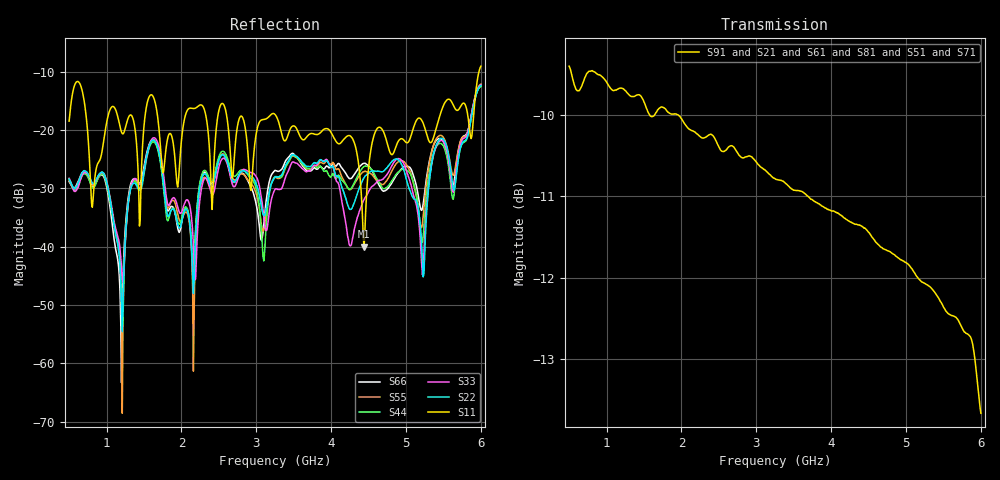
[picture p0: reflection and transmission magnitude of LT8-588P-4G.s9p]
! MTS Systemtechnik GmbH
! S-Parameters
! Model: LT8-588P-6G
! Rohde & Schwarz ZVB8 2Ports - Version 3.20 - 1145.1010k08 SN: 100119
! Converted & adapted with MATLAB
!		|  MTS  |
!		|  |--o OUT 8 (Port 9)
!		|  |--o OUT 7 (Port 8)
!		|  |--o OUT 6 (Port 7)
!		|  |--o OUT 5 (Port 6)
! C (Port 1) o--| LT8-588P-6G |
!		|  |--o OUT 4 (Port 5)
!		|  |--o OUT 3 (Port 4)
!		|  |--o OUT 2 (Port 3)
!		|  |--o OUT 1 (Port 2)
! S9P File: Measurements:
! <S11,S12,S13,S14,S15,S16,S17,S18,S19>,
! <S21,S22,S23,S24,S25,S26,S27,S28,S29>,
! <S31,S32,S33,S34,S35,S36,S37,S38,S39>,
! <S41,S42,S43,S44,S45,S46,S47,S48,S49>,
! <S51,S52,S53,S54,S55,S56,S57,S58,S59>,
! <S61,S62,S63,S64,S65,S66,S67,S68,S69>,
! <S71,S72,S73,S74,S75,S76,S77,S78,S79>,
! <S81,S82,S83,S84,S85,S86,S87,S88,S89>,
! <S91,S92,S93,S94,S95,S96,S97,S98,S99>:
# HZ  S  DB  R  50.00
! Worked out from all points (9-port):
!   551 points, 500 MHz to 6 GHz, reference 50 ohm
!   strongest paths, dB at 500 MHz, 1.87 GHz, 3.25 GHz, 4.63 GHz, 6 GHz:
!     S91: -9.4, -10.0, -10.8, -11.6, -13.7
!     S21: -9.4, -10.0, -10.8, -11.6, -13.8
!     S61: -9.4, -10.0, -10.8, -11.7, -13.7
!     S81: -9.4, -10.0, -10.8, -11.6, -13.8
!     S51: -9.4, -10.0, -10.8, -11.7, -13.8
!     S71: -9.4, -10.0, -10.8, -11.7, -13.7
!   lowest |S11| = -40.0 dB at 4.44 GHz (marker M1), VSWR 1.02, Z = 49.8 + j0.975 ohm
!   |S11| at or under -10 dB: start of sweep to 5.974 GHz
